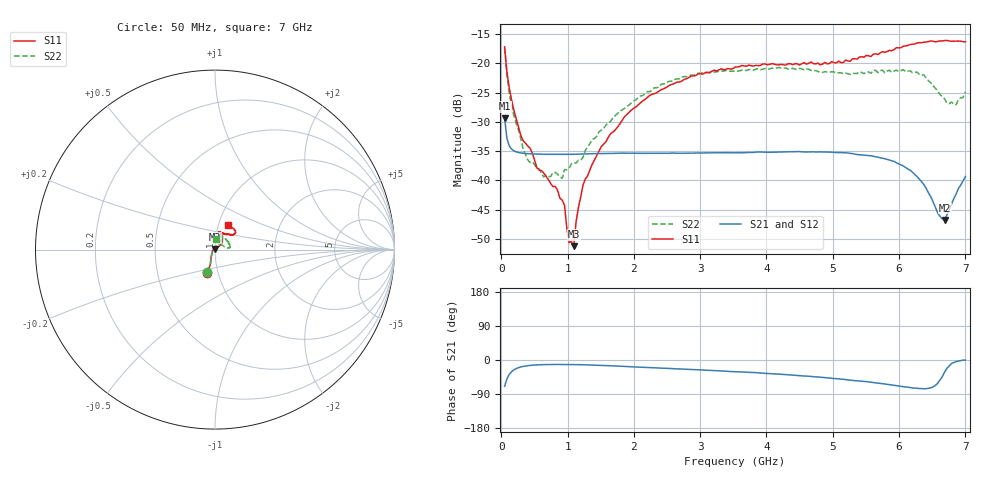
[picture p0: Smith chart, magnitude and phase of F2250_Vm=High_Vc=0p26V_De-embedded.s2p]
! Integrated Device Technology
! Corporate Headquarters
! 6024 Silver Creek Valley Road
! San Jose, CA 95138  USA
! Phone:  1-408-284-8200
! Toll Free:  1-800-223-1366
! Webpage:  http://www.idt.com/
! Timing and RF Division
! 515 Groton Road, Suite 102
! Westford, MA 01886-6024
! Device:  F2250
! Description: Voltage Variable RF Attenuator
! Frequency:  50.0 -  6000.00 MHz
! Package:  3x3 mm Thin QFN Plastic Package: 16 pin
! Ports:  2 RF, 3 DC
!  Pin  1  = GND
!  Pin  2  = NC
!  Pin  3  = RF1  = Port 1
!  Pin  4  = NC
!  Pin  5  = GND
!  Pin  6  = GND
!  Pin  7  = GND
!  Pin  8  = GND
!  Pin  9  = NC
!  Pin 10  = RF2  = Port 2
!  Pin 11  = NC
!  Pin 12  = GND
!  Pin 13  = GND
!  Pin 14  = VCNTRL
!  Pin 15  = VDD
!  Pin 16  = VMODE
! Vcntrl:  0.260 Volts
! Vmode:  +3.300 Volts
! Vdd:  +3.30  Volts
! Current:  1.248 mA
! Data:  The device was measured on a the F2250 evaluation board which has
!  individual transmission lines to the RF pins.  Data was collected
!  using a calibrated network analyzer.  The evaluation board was
!  de-embedded using a TRL calibration technique.
!  The reference plane is the edge of the package pin.
! Misc:  SN 10
!  Action Tracker AT0258
! Date Measured:  2014-11-26
! Date:  2015-10-15  MJV
! Note:
!  Integrated Device Technology supplies this data as a sample of measured
!  data at the package pin for this product.  Your particular data for this
!  product may vary.
!  Data was taken at 25 degrees C.
!  Integrated Device Technology reserves the right to change this data at anytime.
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# GHz S dB R 50
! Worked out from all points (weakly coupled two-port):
!   201 points, 50 MHz to 7 GHz, reference 50 ohm
!   highest |S21| = -29.37 dB at 50 MHz (marker M1); lowest = -46.8 dB at 6.687 GHz (marker M2)
!   lowest |S11| = -51.3 dB at 1.093 GHz (marker M3), VSWR 1.01, Z = 50 + j0.273 ohm
!   |S11| at or under -10 dB: start of sweep to end of sweep
!   |S22| runs from -39.7 to -17.4 dB; largest |S21 - S12| = 5.9e-05
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0.05  -17.18 -108.5  -29.37 -69.4  -29.37 -69.4  -17.40 -110.4
0.08475  -21.47 -107.4  -32.84 -50.0  -32.84 -50.0  -21.93 -108.7
0.15425  -26.23 -116.5  -34.66 -31.0  -34.66 -30.9  -27.20 -119.9
0.29325  -32.27 -127.5  -35.32 -18.4  -35.33 -18.4  -32.85 -132.3
0.3975  -34.11 -142.2  -35.45 -15.0  -35.45 -15.0  -36.47 -157.2
0.5365  -37.86 -154.7  -35.53 -12.9  -35.53 -12.9  -37.95 -179.5
0.64075  -38.77 -162.5  -35.55 -12.2  -35.55 -12.2  -39.42 160.0
0.91875  -43.41 156.0  -35.58 -11.8  -35.58 -11.8  -39.67 125.4
0.9535  -44.27 170.9  -35.57 -11.8  -35.58 -11.8  -38.17 122.1
1.023  -50.67 140.9  -35.57 -11.9  -35.57 -11.9  -37.97 105.4
1.0925  -51.26 88.8  -35.55 -12.0  -35.55 -12.0  -37.01 96.1
1.12725  -47.18 61.5  -35.54 -12.1  -35.54 -12.1  -37.06 89.0
1.2315  -40.86 41.0  -35.50 -12.5  -35.50 -12.5  -36.10 74.8
1.6485  -32.03 41.3  -35.41 -15.2  -35.41 -15.2  -29.91 58.8
2.37825  -24.75 46.7  -35.37 -21.1  -35.38 -21.1  -24.03 53.3
3.525  -20.65 71.7  -35.30 -30.6  -35.30 -30.7  -21.31 72.6
4.7065  -20.06 72.0  -35.13 -44.0  -35.14 -44.0  -21.27 70.1
5.85325  -17.79 40.5  -36.56 -64.9  -36.56 -65.1  -21.17 23.1
6.27025  -16.53 39.4  -39.35 -74.6  -39.37 -74.6  -21.49 8.3
6.68725  -16.11 47.9  -46.76 -31.6  -46.73 -31.3  -26.10 28.2
6.861  -16.22 54.5  -42.31 -4.1  -42.27 -4.1  -27.06 57.4
7  -16.32 62.4  -39.36 -0.4  -39.32 -0.6  -24.87 83.8
